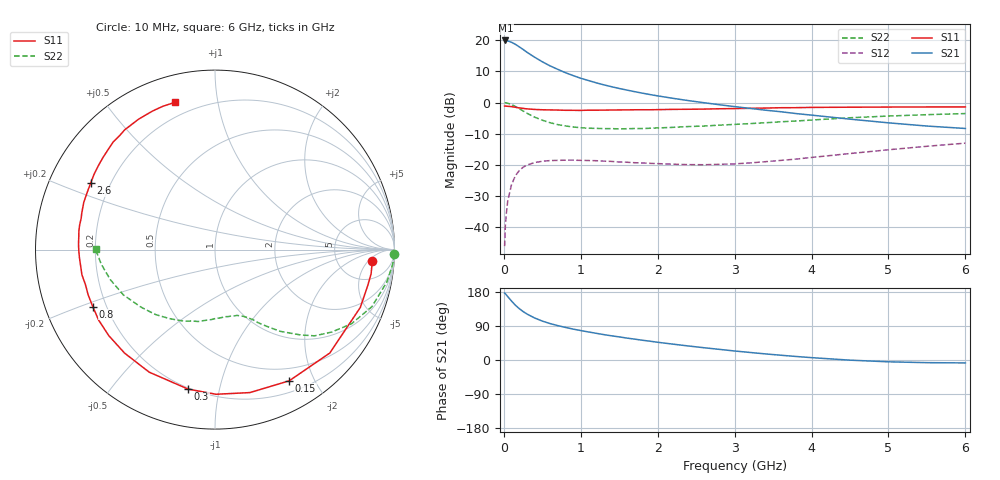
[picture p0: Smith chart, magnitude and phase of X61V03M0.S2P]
! SIEMENS Small Signal Semiconductors
! BFP193W
! Si NPN RF Bipolar Junction Transistor in SOT343
! VCE = 1 V  IC = 3 mA
! Common Emitter S-Parameters:  April 1994
# GHz  S  MA  R  50
!  f  S11  S21  S12  S22
! GHz  MAG  ANG  MAG  ANG  MAG  ANG  MAG  ANG
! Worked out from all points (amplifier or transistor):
!   40 points, 10 MHz to 6 GHz, reference 50 ohm
!   highest |S21| = 20.0 dB at 20 MHz (marker M1)
!   |S21| within 3 dB of that: start of sweep to 256.3 MHz
!   unconditionally stable (mu >= 1): 1.856 GHz to end of sweep
!   at 200 MHz: K = 0.11, MSG = 19.9 dB, |S12| = -21.9 dB
!   at 1.5 GHz: K = 0.80, MSG = 11.8 dB, |S12| = -19.1 dB
!   at 6 GHz: K = 1.05, MAG = 0.9 dB, |S12| = -13.1 dB
!   S11 on the Smith chart (normalised r, x): 10 MHz: 12, -7; 150 MHz: 0.34, -1.66; 300 MHz: 0.19, -0.81; 800 MHz: 0.15, -0.22; 2.6 GHz: 0.13, +0.25; 6 GHz: 0.13, +0.76
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0.01  0.8787 -4.3  9.916 176.7  0.0049 86.8  0.999 -1.4
0.02  0.8802 -8.8  9.975 175.0  0.0106 84.9  0.9938 -4.4
0.05  0.8714 -21.7  9.83 167.5  0.0258 78.1  0.9748 -10.6
0.1  0.8609 -42.0  9.325 155.6  0.048 67.7  0.9301 -20.0
0.15  0.8399 -60.5  8.651 144.6  0.0665 58.1  0.8657 -28.5
0.2  0.82 -76.3  7.874 135.6  0.0805 50.3  0.7966 -35.2
0.25  0.806 -89.6  7.154 128.0  0.0911 43.7  0.7338 -40.9
0.3  0.7916 -100.9  6.453 121.4  0.0988 38.5  0.6738 -44.9
0.4  0.775 -118.2  5.365 110.9  0.1084 30.2  0.5827 -51.4
0.5  0.7658 -131.1  4.531 102.7  0.1137 24.7  0.5198 -55.7
0.6  0.7616 -141.0  3.895 96.2  0.1166 20.4  0.4747 -59.3
0.7  0.758 -148.8  3.426 90.8  0.1176 17.5  0.4422 -61.7
0.8  0.7515 -155.0  3.026 86.0  0.1184 15.0  0.4207 -64.4
1.1  0.7546 -169.2  2.261 74.0  0.1169 10.4  0.3865 -71.5
1.3  0.7565 -176.4  1.927 67.0  0.1142 8.6  0.3809 -76.4
1.6  0.7622 174.7  1.588 57.8  0.1097 8.4  0.3797 -83.4
2.2  0.777 160.3  1.169 41.8  0.1019 12.2  0.3992 -98.4
2.6  0.7855 151.9  0.995 32.4  0.1 17.7  0.419 -108.4
3.2  0.8082 140.5  0.806 19.9  0.107 27.1  0.4588 -122.9
4.5  0.8422 120.3  0.541 -0.4  0.1514 37.2  0.5696 -153.7
5.5  0.8498 109.9  0.419 -7.0  0.198 35.5  0.6385 -172.6
6  0.8501 105.1  0.383 -7.7  0.2225 33.4  0.6656 179.9
